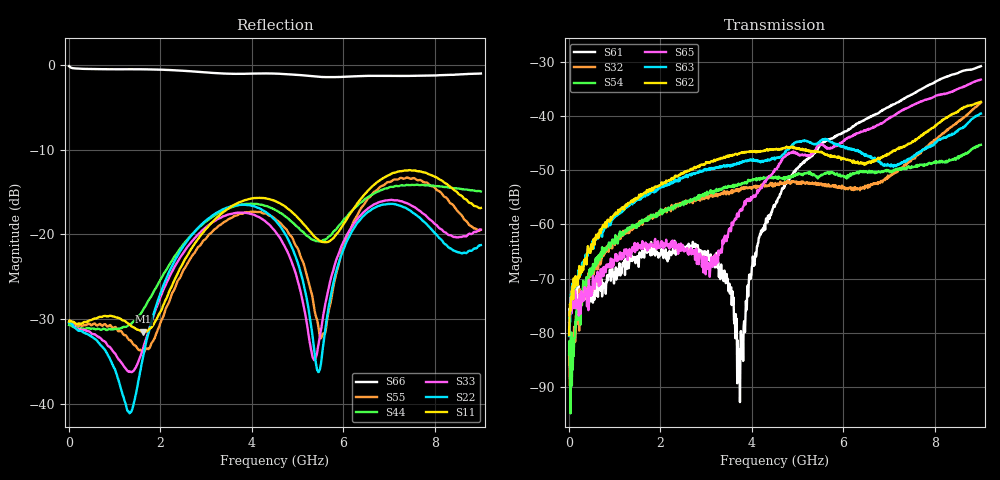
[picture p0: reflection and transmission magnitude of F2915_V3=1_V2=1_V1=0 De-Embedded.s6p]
! Integrated Device Technology
! Corporate Headquarters
! 6024 Silver Creek Valley Road
! San Jose, CA 95138  USA
! Phone:  1-408-284-8200
! Toll Free:  1-800-223-1366
! Webpage:  http://www.idt.com/
! Timing and RF Division
! 515 Groton Road, Suite 102
! Westford, MA 01886-6024
! Device:  F2915
! Description: High Reliability SP5T RF Switch
! Frequency:  0.05 -  8.GHz
! Package:  4x4 mm Thin QFN Plastic Package: 24 pin
! Ports:  6 RF,  5 DC
!  Pin  1  = GND
!  Pin  2  = RF5  =  Port 5
!  Pin  3  = GND
!  Pin  4  = GND
!  Pin  5  = RF4  =  Port 4
!  Pin  6  = GND
!  Pin  7  = GND
!  Pin  8  = RF3  =  Port 3
!  Pin  9  = GND
!  Pin 10  = GND
!  Pin 11  = RF2  =  Port 2
!  Pin 12  = GND
!  Pin 13  = GND
!  Pin 14  = RF1  =  Port 1
!  Pin 15  = GND
!  Pin 16  = Vcc
!  Pin 17  = V1
!  Pin 18  = V2
!  Pin 19  = V3
!  Pin 20  = VSSext
!  Pin 21  = GND
!  Pin 22  = RFC  =  Port 6
!  Pin 23  = GND
!  Pin 24  = GND
! Voltage:  VDD  =  +3.30 Volts
!  VSSEXT =  0.00 Volts
! Current:  IDD  = 275  uA
! State:  All OFF
! V1:  Logic LOW
! V2:  Logic HIGH
! V3:  Logic HIGH
! Data:  The device was measured on the F291x evaluation board which has
!  individual transmission lines to the RF pins.  Data was collected
!  using a calibrated network analyzer.  The input lines were
!  modeled using Automatic Fixture Removal (AFR) from Keysight.
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# Hz S  dB  R 50
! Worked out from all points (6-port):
!   900 points, 10 MHz to 9 GHz, reference 50 ohm
!   strongest paths, dB at 10 MHz, 2.26 GHz, 4.51 GHz, 6.76 GHz, 9 GHz:
!     S62: -80.4, -51.4, -46.1, -47.7, -37.4
!     S63: -80.6, -52.2, -47.8, -48.3, -39.5
!     S65: -78.0, -64.0, -49.8, -41.7, -33.3
!     S54: -84.0, -57.0, -51.3, -50.2, -45.3
!     S32: -83.4, -56.8, -52.4, -52.2, -37.6
!     S61: -79.6, -65.1, -56.3, -39.5, -30.8
!   lowest |S11| = -31.5 dB at 1.63 GHz (marker M1), VSWR 1.05, Z = 49.6 + j2.62 ohm
!   |S11| at or under -10 dB: start of sweep to end of sweep
